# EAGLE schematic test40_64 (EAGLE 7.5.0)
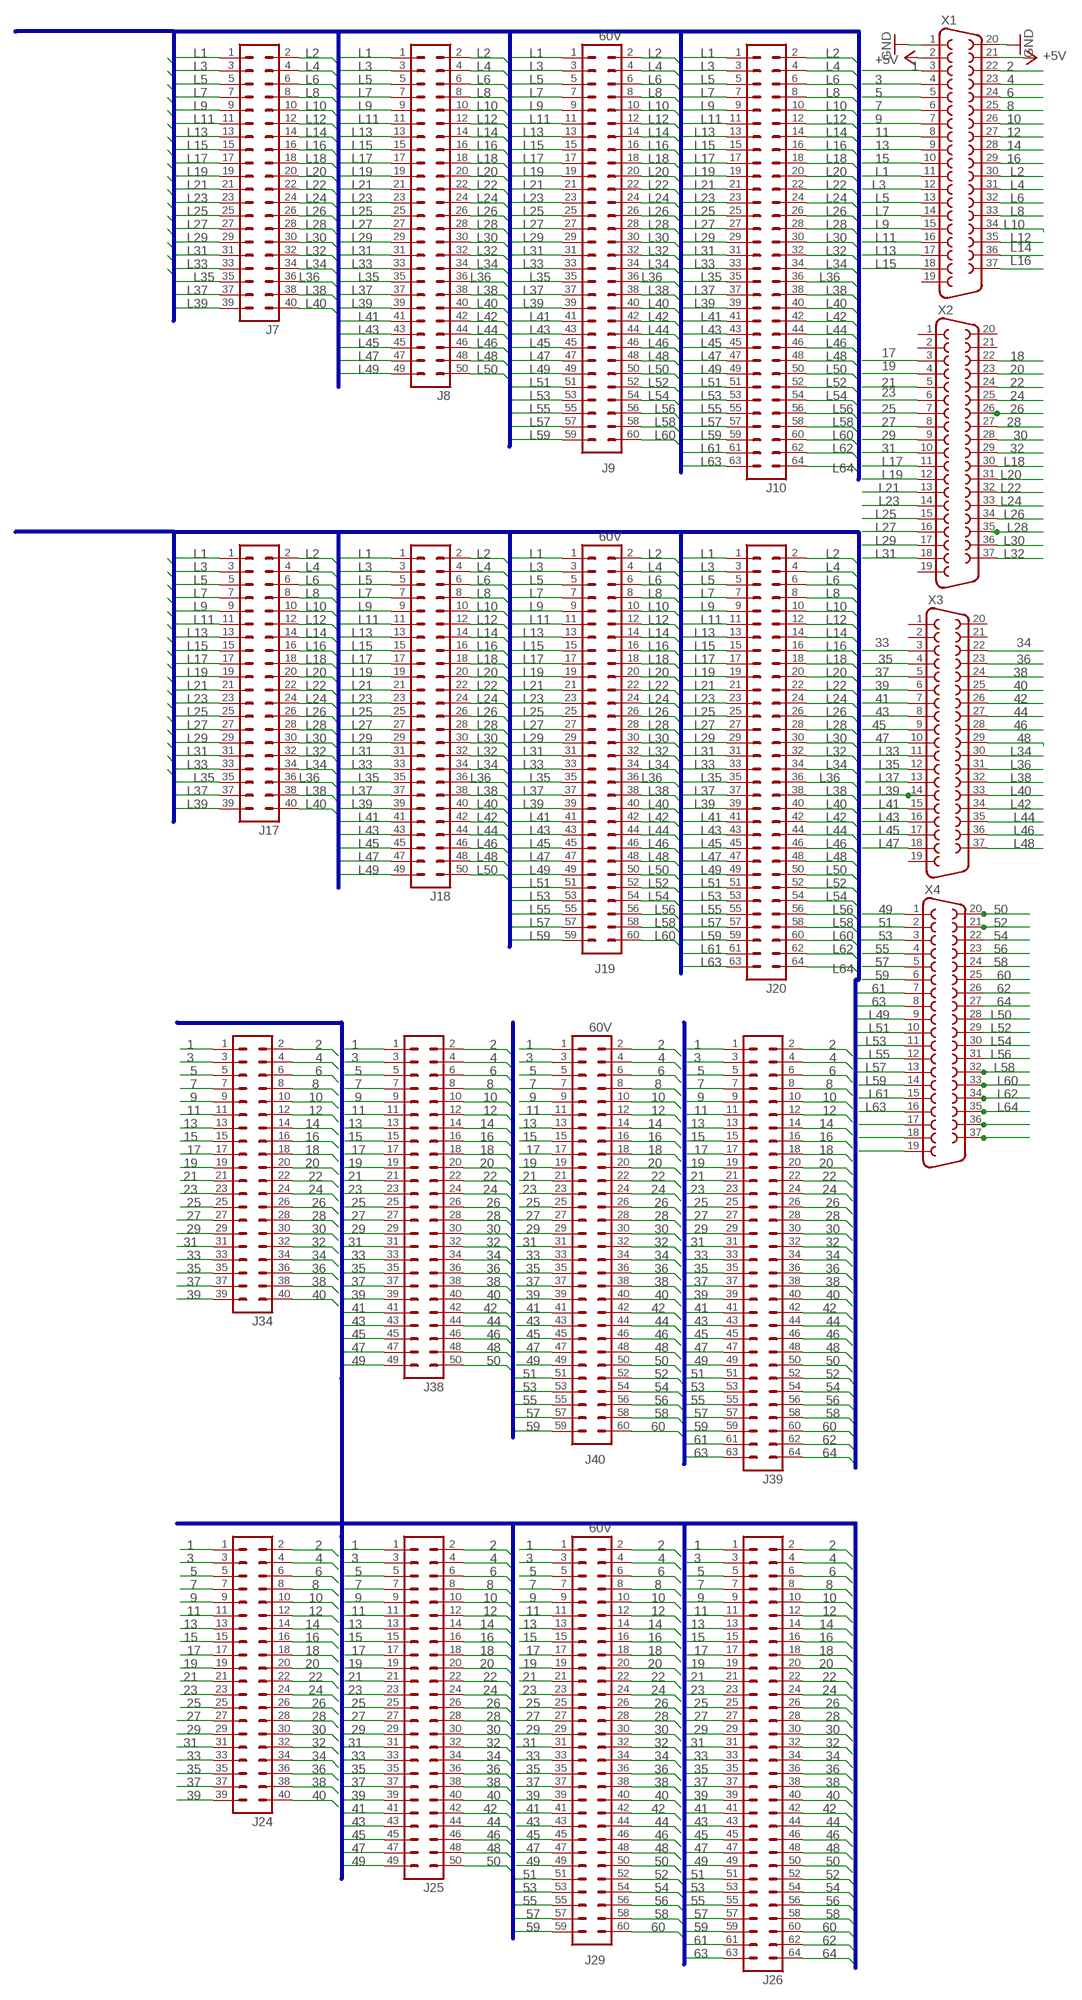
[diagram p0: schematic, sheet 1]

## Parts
J7  40V  [40V]
J8  50V  [50V]
J9  60V  [60V]
J10  64V  [64V]
J17  40V  [40V]
J18  50V  [50V]
J19  60V  [60V]
J20  64V  [64V]
J24  40V  [40V]
J25  50V  [50V]
J26  64V  [64V]
J29  60V  [60V]
J34  40V  [40V]
J38  50V  [50V]
J39  64V  [64V]
J40  60V  [60V]
X1  F37V  [F37V]
X2  F37V  [F37V]
X3  F37V  [F37V]
X4  F37V  [F37V]

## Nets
1: J24.1 J25.1 J26.1 J29.1 J34.1 J38.1 J39.1 J40.1 X1.3
2: J24.2 J25.2 J26.2 J29.2 J34.2 J38.2 J39.2 J40.2 X1.22
3: J24.3 J25.3 J26.3 J29.3 J34.3 J38.3 J39.3 J40.3 X1.4
4: J24.4 J25.4 J26.4 J29.4 J34.4 J38.4 J39.4 J40.4 X1.23
5: J24.5 J25.5 J26.5 J29.5 J34.5 J38.5 J39.5 J40.5 X1.5
6: J24.6 J25.6 J26.6 J29.6 J34.6 J38.6 J39.6 J40.6 X1.24
7: J24.7 J25.7 J26.7 J29.7 J34.7 J38.7 J39.7 J40.7 X1.6
8: J24.8 J25.8 J26.8 J29.8 J34.8 J38.8 J39.8 J40.8 X1.25
9: J24.9 J25.9 J26.9 J29.9 J34.9 J38.9 J39.9 J40.9 X1.7
10: J24.10 J25.10 J26.10 J29.10 J34.10 J38.10 J39.10 J40.10 X1.26
11: J24.11 J25.11 J26.11 J29.11 J34.11 J38.11 J39.11 J40.11 X1.8
12: J24.12 J25.12 J26.12 J29.12 J34.12 J38.12 J39.12 J40.12 X1.27
13: J24.13 J25.13 J26.13 J29.13 J34.13 J38.13 J39.13 J40.13 X1.9
14: J24.14 J25.14 J26.14 J29.14 J34.14 J38.14 J39.14 J40.14 X1.28
15: J24.15 J25.15 J26.15 J29.15 J34.15 J38.15 J39.15 J40.15 X1.10
16: J24.16 J25.16 J26.16 J29.16 J34.16 J38.16 J39.16 J40.16 X1.29
17: J24.17 J25.17 J26.17 J29.17 J34.17 J38.17 J39.17 J40.17 X2.3
18: J24.18 J25.18 J26.18 J29.18 J34.18 J38.18 J39.18 J40.18 X2.22
19: J24.19 J25.19 J26.19 J29.19 J34.19 J38.19 J39.19 J40.19 X2.4
20: J24.20 J25.20 J26.20 J29.20 J34.20 J38.20 J39.20 J40.20 X2.23
21: J24.21 J25.21 J26.21 J29.21 J34.21 J38.21 J39.21 J40.21 X2.5
22: J24.22 J25.22 J26.22 J29.22 J34.22 J38.22 J39.22 J40.22 X2.24
23: J24.23 J25.23 J26.23 J29.23 J34.23 J38.23 J39.23 J40.23 X2.6
24: J24.24 J25.24 J26.24 J29.24 J34.24 J38.24 J39.24 J40.24 X2.25
25: J24.25 J25.25 J26.25 J29.25 J34.25 J38.25 J39.25 J40.25 X2.7
26: J24.26 J25.26 J26.26 J29.26 J34.26 J38.26 J39.26 J40.26 X2.26
27: J24.27 J25.27 J26.27 J29.27 J34.27 J38.27 J39.27 J40.27 X2.8
28: J24.28 J25.28 J26.28 J29.28 J34.28 J38.28 J39.28 J40.28 X2.27
29: J24.29 J25.29 J26.29 J29.29 J34.29 J38.29 J39.29 J40.29 X2.9
30: J24.30 J25.30 J26.30 J29.30 J34.30 J38.30 J39.30 J40.30 X2.28
31: J24.31 J25.31 J26.31 J29.31 J34.31 J38.31 J39.31 J40.31 X2.10
32: J24.32 J25.32 J26.32 J29.32 J34.32 J38.32 J39.32 J40.32 X2.29
33: J24.33 J25.33 J26.33 J29.33 J34.33 J38.33 J39.33 J40.33 X3.3
34: J24.34 J25.34 J26.34 J29.34 J34.34 J38.34 J39.34 J40.34 X3.22
35: J24.35 J25.35 J26.35 J29.35 J34.35 J38.35 J39.35 J40.35 X3.4
36: J24.36 J25.36 J26.36 J29.36 J34.36 J38.36 J39.36 J40.36 X3.23
37: J24.37 J25.37 J26.37 J29.37 J34.37 J38.37 J39.37 J40.37 X3.5
38: J24.38 J25.38 J26.38 J29.38 J34.38 J38.38 J39.38 J40.38 X3.24
39: J24.39 J25.39 J26.39 J29.39 J34.39 J38.39 J39.39 J40.39 X3.6
40: J24.40 J25.40 J26.40 J29.40 J34.40 J38.40 J39.40 J40.40 X3.25
41: J25.41 J26.41 J29.41 J38.41 J39.41 J40.41 X3.7
42: J25.42 J26.42 J29.42 J38.42 J39.42 J40.42 X3.26
43: J25.43 J26.43 J29.43 J38.43 J39.43 J40.43 X3.8
44: J25.44 J26.44 J29.44 J38.44 J39.44 J40.44 X3.27
45: J25.45 J26.45 J29.45 J38.45 J39.45 J40.45 X3.9
46: J25.46 J26.46 J29.46 J38.46 J39.46 J40.46 X3.28
47: J25.47 J26.47 J29.47 J38.47 J39.47 J40.47 X3.10
48: J25.48 J26.48 J29.48 J38.48 J39.48 J40.48 X3.29
49: J25.49 J26.49 J29.49 J38.49 J39.49 J40.49 X4.1
50: J25.50 J26.50 J29.50 J38.50 J39.50 J40.50 X4.20
51: J26.51 J29.51 J39.51 J40.51 X4.2
52: J26.52 J29.52 J39.52 J40.52 X4.21
53: J26.53 J29.53 J39.53 J40.53 X4.3
54: J26.54 J29.54 J39.54 J40.54 X4.22
55: J26.55 J29.55 J39.55 J40.55 X4.4
56: J26.56 J29.56 J39.56 J40.56 X4.23
57: J26.57 J29.57 J39.57 J40.57 X4.5
58: J26.58 J29.58 J39.58 J40.58 X4.24
59: J26.59 J29.59 J39.59 J40.59 X4.6
60: J26.60 J29.60 J39.60 J40.60 X4.25
61: J26.61 J39.61 X4.7
62: J26.62 J39.62 X4.26
63: J26.63 J39.63 X4.8
64: J26.64 J39.64 X4.27
+5V: X1.2 X1.21
GND: X1.1 X1.20
L1: J7.1 J8.1 J9.1 J10.1 J17.1 J18.1 J19.1 J20.1 X1.11
L2: J7.2 J8.2 J9.2 J10.2 J17.2 J18.2 J19.2 J20.2 X1.30
L3: J7.3 J8.3 J9.3 J10.3 J17.3 J18.3 J19.3 J20.3 X1.12
L4: J7.4 J8.4 J9.4 J10.4 J17.4 J18.4 J19.4 J20.4 X1.31
L5: J7.5 J8.5 J9.5 J10.5 J17.5 J18.5 J19.5 J20.5 X1.13
L6: J7.6 J8.6 J9.6 J10.6 J17.6 J18.6 J19.6 J20.6 X1.32
L7: J7.7 J8.7 J9.7 J10.7 J17.7 J18.7 J19.7 J20.7 X1.14
L8: J7.8 J8.8 J9.8 J10.8 J17.8 J18.8 J19.8 J20.8 X1.33
L9: J7.9 J8.9 J9.9 J10.9 J17.9 J18.9 J19.9 J20.9 X1.15
L10: J7.10 J8.10 J9.10 J10.10 J17.10 J18.10 J19.10 J20.10 X1.34
L11: J7.11 J8.11 J9.11 J10.11 J17.11 J18.11 J19.11 J20.11 X1.16
L12: J7.12 J8.12 J9.12 J10.12 J17.12 J18.12 J19.12 J20.12 X1.35
L13: J7.13 J8.13 J9.13 J10.13 J17.13 J18.13 J19.13 J20.13 X1.17
L14: J7.14 J8.14 J9.14 J10.14 J17.14 J18.14 J19.14 J20.14 X1.36
L15: J7.15 J8.15 J9.15 J10.15 J17.15 J18.15 J19.15 J20.15 X1.18
L16: J7.16 J8.16 J9.16 J10.16 J17.16 J18.16 J19.16 J20.16 X1.37
L17: J7.17 J8.17 J9.17 J10.17 J17.17 J18.17 J19.17 J20.17 X2.11
L18: J7.18 J8.18 J9.18 J10.18 J17.18 J18.18 J19.18 J20.18 X2.30
L19: J7.19 J8.19 J9.19 J10.19 J17.19 J18.19 J19.19 J20.19 X2.12
L20: J7.20 J8.20 J9.20 J10.20 J17.20 J18.20 J19.20 J20.20 X2.31
L21: J7.21 J8.21 J9.21 J10.21 J17.21 J18.21 J19.21 J20.21 X2.13
L22: J7.22 J8.22 J9.22 J10.22 J17.22 J18.22 J19.22 J20.22 X2.32
L23: J7.23 J8.23 J9.23 J10.23 J17.23 J18.23 J19.23 J20.23 X2.14
L24: J7.24 J8.24 J9.24 J10.24 J17.24 J18.24 J19.24 J20.24 X2.33
L25: J7.25 J8.25 J9.25 J10.25 J17.25 J18.25 J19.25 J20.25 X2.15
L26: J7.26 J8.26 J9.26 J10.26 J17.26 J18.26 J19.26 J20.26 X2.34
L27: J7.27 J8.27 J9.27 J10.27 J17.27 J18.27 J19.27 J20.27 X2.16
L28: J7.28 J8.28 J9.28 J10.28 J17.28 J18.28 J19.28 J20.28 X2.35
L29: J7.29 J8.29 J9.29 J10.29 J17.29 J18.29 J19.29 J20.29 X2.17
L30: J7.30 J8.30 J9.30 J10.30 J17.30 J18.30 J19.30 J20.30 X2.36
L31: J7.31 J8.31 J9.31 J10.31 J17.31 J18.31 J19.31 J20.31 X2.18
L32: J7.32 J8.32 J9.32 J10.32 J17.32 J18.32 J19.32 J20.32 X2.37
L33: J7.33 J8.33 J9.33 J10.33 J17.33 J18.33 J19.33 J20.33 X3.11
L34: J7.34 J8.34 J9.34 J10.34 J17.34 J18.34 J19.34 J20.34 X3.30
L35: J7.35 J8.35 J9.35 J10.35 J17.35 J18.35 J19.35 J20.35 X3.12
L36: J7.36 J8.36 J9.36 J10.36 J17.36 J18.36 J19.36 J20.36 X3.31
L37: J7.37 J8.37 J9.37 J10.37 J17.37 J18.37 J19.37 J20.37 X3.13
L38: J7.38 J8.38 J9.38 J10.38 J17.38 J18.38 J19.38 J20.38 X3.32
L39: J7.39 J8.39 J9.39 J10.39 J17.39 J18.39 J19.39 J20.39 X3.14
L40: J7.40 J8.40 J9.40 J10.40 J17.40 J18.40 J19.40 J20.40 X3.33
L41: J8.41 J9.41 J10.41 J18.41 J19.41 J20.41 X3.15
L42: J8.42 J9.42 J10.42 J18.42 J19.42 J20.42 X3.34
L43: J8.43 J9.43 J10.43 J18.43 J19.43 J20.43 X3.16
L44: J8.44 J9.44 J10.44 J18.44 J19.44 J20.44 X3.35
L45: J8.45 J9.45 J10.45 J18.45 J19.45 J20.45 X3.17
L46: J8.46 J9.46 J10.46 J18.46 J19.46 J20.46 X3.36
L47: J8.47 J9.47 J10.47 J18.47 J19.47 J20.47 X3.18
L48: J8.48 J9.48 J10.48 J18.48 J19.48 J20.48 X3.37
L49: J8.49 J9.49 J10.49 J18.49 J19.49 J20.49 X4.9
L50: J8.50 J9.50 J10.50 J18.50 J19.50 J20.50 X4.28
L51: J9.51 J10.51 J19.51 J20.51 X4.10
L52: J9.52 J10.52 J19.52 J20.52 X4.29
L53: J9.53 J10.53 J19.53 J20.53 X4.11
L54: J9.54 J10.54 J19.54 J20.54 X4.30
L55: J9.55 J10.55 J19.55 J20.55 X4.12
L56: J9.56 J10.56 J19.56 J20.56 X4.31
L57: J9.57 J10.57 J19.57 J20.57 X4.13
L58: J9.58 J10.58 J19.58 J20.58 X4.32
L59: J9.59 J10.59 J19.59 J20.59 X4.14
L60: J9.60 J10.60 J19.60 J20.60 X4.33
L61: J10.61 J20.61 X4.15
L62: J10.62 J20.62 X4.34
L63: J10.63 J20.63 X4.16
L64: J10.64 J20.64 X4.35
N$17: X4.17
N$18: X4.18
N$19: X4.19
N$37: X4.36
N$38: X4.37
Unconnected: X1.19 X2.1 X2.2 X2.19 X2.20 X2.21 X3.1 X3.2 X3.19 X3.20 X3.21

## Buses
B$1

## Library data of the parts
J7 J17 J24 J34 = con-harting-v:40V: CONNECTOR; OC_FARNELL: unknown; OC_NEWARK: unknown
J8 J18 J25 J38 = con-harting-v:50V: CONNECTOR; OC_FARNELL: unknown; OC_NEWARK: unknown
J9 J19 J29 J40 = con-harting-v:60V
J10 J20 J26 J39 = con-harting-v:64V: CONNECTOR; OC_FARNELL: unknown; OC_NEWARK: unknown
X1-X4 = con-subd:F37: SUB-D; OC_FARNELL: unknown; OC_NEWARK: unknown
